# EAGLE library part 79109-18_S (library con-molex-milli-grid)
RECEPTACAL
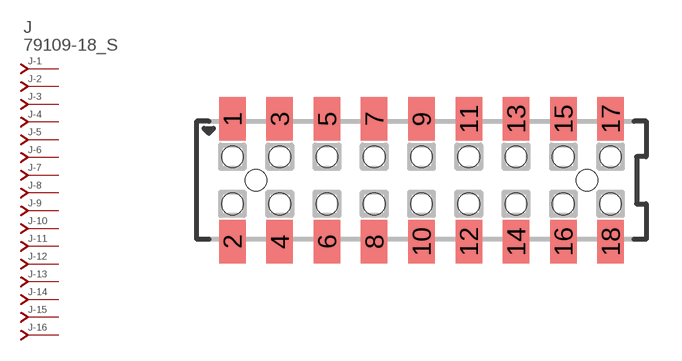
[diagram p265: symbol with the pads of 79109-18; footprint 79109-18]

Designator prefix J; gates -1=J-NV -2=J-N -3=J-N -4=J-N -5=J-N -6=J-N -7=J-N -8=J-N -9=J-N -10=J-N -11=J-N -12=J-N -13=J-N -14=J-N -15=J-N -16=J-N -17=J-N -18=J-N

## 79109-18_S  [79109-18]
1  -1:J  pas
2  -2:J  pas
3  -3:J  pas
4  -4:J  pas
5  -5:J  pas
6  -6:J  pas
7  -7:J  pas
8  -8:J  pas
9  -9:J  pas
10  -10:J  pas
11  -11:J  pas
12  -12:J  pas
13  -13:J  pas
14  -14:J  pas
15  -15:J  pas
16  -16:J  pas
17  -17:J  pas
18  -18:J  pas

## Footprint 79109-18 (pad centres in mm)
RECEPTACAL SMD Dual Row, Vertical, Pass-Thru
smd 1.12 x 1.83: 1 -8,2.6; 2 -8,-2.6; 3 -6,2.6; 4 -6,-2.6; 5 -4,2.6; 6 -4,-2.6; 7 -2,2.6; 8 -2,-2.6; 9 0,2.6; 10 0,-2.6; 11 2,2.6; 12 2,-2.6; 13 4,2.6; 14 4,-2.6; 15 6,2.6; 16 6,-2.6; 17 8,2.6; 18 8,-2.6
hole 0.914 at -7,0
hole 0.914 at -8,1
hole 0.914 at -8,-1
hole 0.914 at -6,-1
hole 0.914 at -6,1
hole 0.914 at -4,-1
hole 0.914 at -4,1
hole 0.914 at 7,0
hole 0.914 at -2,1
hole 0.914 at -2,-1
hole 0.914 at 0,1
hole 0.914 at 0,-1
hole 0.914 at 2,1
hole 0.914 at 2,-1
hole 0.914 at 4,1
hole 0.914 at 4,-1
hole 0.914 at 6,-1
hole 0.914 at 6,1
hole 0.914 at 8,1
hole 0.914 at 8,-1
